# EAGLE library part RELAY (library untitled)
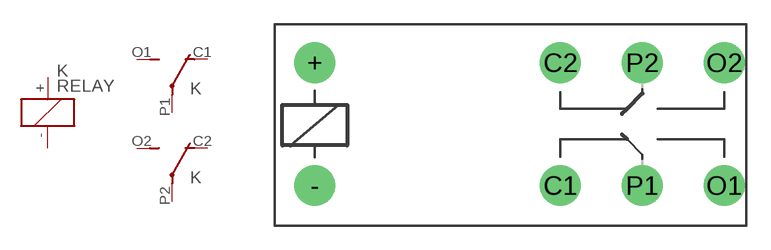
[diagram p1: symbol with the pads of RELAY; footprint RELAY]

Designator prefix K; gates G$1=CON G$2=CON G$3=REL

## RELAY  [RELAY]
+  G$3:+  pas
-  G$3:-  pas
C1  G$1:C  pas
C2  G$2:C  pas
O1  G$1:O  pas
O2  G$2:O  pas
P1  G$1:P  pas
P2  G$2:P  pas

## Footprint RELAY (pad centres in mm)
drill 0.5 pad 2.54: + -10.795,3.81; - -10.795,-3.81; C1 4.445,-3.81; C2 4.445,3.81; O1 14.605,-3.81; O2 14.605,3.81; P1 9.525,-3.81; P2 9.525,3.81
